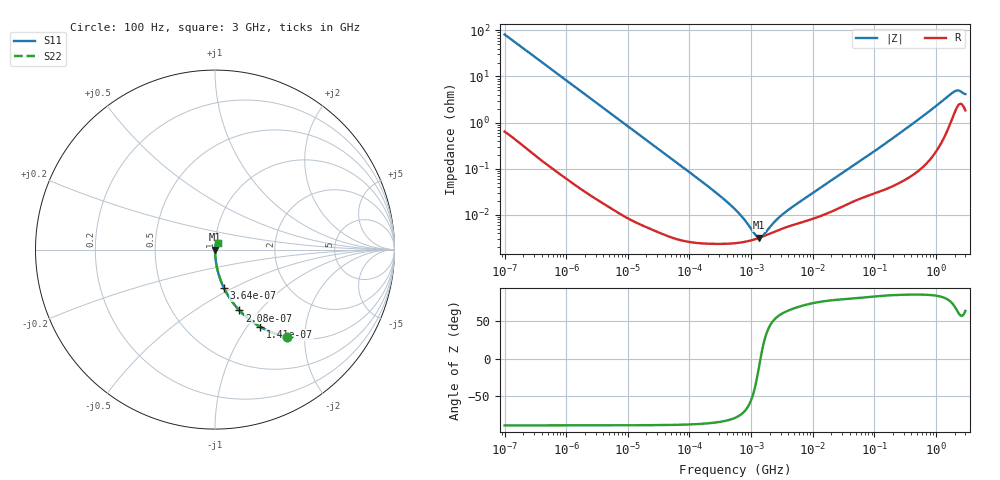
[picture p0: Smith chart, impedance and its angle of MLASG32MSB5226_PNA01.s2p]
! MLASG32MSB5226_PNA01  S-PARAMETER MODEL  ( Standard Model )
! Model Generated by TAIYO YUDEN Corporation (http://www.ty-top.com)
! Version 1.0
! TAIYO YUDEN Control No. 220601
! Copyright(c) 2013 TAIYO YUDEN CO.,LTD. All Rights Reserved.
! Product Description (link to TY-COMPAS)
! https://ds.yuden.co.jp/TYCOMPAS/or/detail?pn=MLASG32MSB5226MPNA01&u=M
! Products Name : Multilayer Ceramic Capacitors
! Characteristics :
!  Capacitance : 22 [uF] , Rated Voltage : 35 [V] , TCC : X5R
!  Case Size : 3.2 x 2.5 / 0.126 x 0.098 [mm/inch] , Thickness : 2.5 / 0.098 [mm/inch]
!  (Conditions: Temperature = 25 [degC] , DC Bias Voltage = 0 [V])
! External Node Assignments :
!  1  o---| |---o  2
! GND o---------o GND
! Frequency Range : 100Hz  -  3GHz  [ 401 STEP ]
# MHZ S RI R 50
! Freq[MHz].  S11 Real  S11 Imag  S21 Real  S21 Imag  S12 Real  S12 Imag  S22 Real  S22 Imag
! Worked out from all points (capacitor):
!   401 points, 100 Hz to 3 GHz, reference 50 ohm
!   read as one part in series: C = 19.5 uF near 109 Hz
!   lowest |Z| = 3.21 mohm at 1.352 MHz (marker M1)
!   series resonance near 1.422 MHz, so ESL is about 640 pH
!   S11 on the Smith chart (normalised r, x): 100 Hz: 1.01, -1.63; 141 Hz: 1.01, -1.16; 208 Hz: 1.01, -0.79; 364 Hz: 1.00, -0.45; 3 GHz: 1.04, +0.07
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0.0001  0.3997 -0.4859  0.6003 0.4859  0.6003 0.4859  0.3997 -0.4859
0.000141  0.2524 -0.4305  0.7476 0.4305  0.7476 0.4305  0.2524 -0.4305
0.000208  0.136 -0.339  0.864 0.339  0.864 0.339  0.136 -0.339
0.000364  0.0498 -0.2139  0.9502 0.2139  0.9502 0.2139  0.0498 -0.2139
0.000756  0.0125 -0.1074  0.9875 0.1074  0.9875 0.1074  0.0125 -0.1074
0.001788  0.00248 -0.0461  0.9975 0.0461  0.9975 0.0461  0.00248 -0.0461
0.005476  0.000364 -0.0152  0.9996 0.0152  0.9996 0.0152  0.000364 -0.0152
0.031977  4.79e-05 -0.00262  1 0.00262  1 0.00262  4.79e-05 -0.00262
0.231582  2.35e-05 -0.000353  1 0.000353  1 0.000353  2.35e-05 -0.000353
0.371814  2.34e-05 -0.00021  1 0.00021  1 0.00021  2.34e-05 -0.00021
0.547723  2.41e-05 -0.00013  1 0.00013  1 0.00013  2.41e-05 -0.00013
0.623217  2.46e-05 -0.000108  1 0.000108  1 0.000108  2.46e-05 -0.000108
0.709116  2.52e-05 -8.75e-05  1 8.75e-05  1 8.75e-05  2.52e-05 -8.75e-05
1.352413  3.16e-05 -5.54e-06  1 5.54e-06  1 5.54e-06  3.16e-05 -5.54e-06
3.198641  4.99e-05 8.74e-05  1 -8.74e-05  1 -8.74e-05  4.99e-05 8.74e-05
9.794414  8.08e-05 0.00028  0.9999 -0.00028  0.9999 -0.00028  8.08e-05 0.00028
175.1444  0.000402 0.00403  0.9996 -0.00403  0.9996 -0.00403  0.000402 0.00403
610.2215  0.00126 0.0137  0.9987 -0.0137  0.9987 -0.0137  0.00126 0.0137
1868.531  0.0146 0.0416  0.9854 -0.0416  0.9854 -0.0416  0.0146 0.0416
2126.076  0.0213 0.0432  0.9787 -0.0432  0.9787 -0.0432  0.0213 0.0432
2317.205  0.0253 0.0414  0.9747 -0.0414  0.9747 -0.0414  0.0253 0.0414
3000  0.0193 0.0358  0.9807 -0.0358  0.9807 -0.0358  0.0193 0.0358
